| IBS file for GS832xxxxxA
| Package: standard 209pin BGA
| DQ driver is programmable
| VDD=3.3V, VDDQ can be either 2.5V or 3.3V
| Date:   23 August 2006
| Rev.:
[IBIS Ver]   3.2
[File name]   gs832xxxxxa.ibs
[File Rev]   1.0
[Date]   08/23/06
[Component]   GS832018T
[Manufacturer]   GSI Technology
[Package]
|  variable   typ   min   max
R_pkg   0.2   0.1   0.5
L_pkg   3nH   1nH   5nH
C_pkg   1.5pF   1pF   3pF
[Pin]   signal_name model_name  R_pin   L_pin   C_pin
 1   NC   NC
 2   NC   NC
 3   NC   NC
 4   VDDQ   POWER
 5   VSS   GND
 6   NC   NC
 7   NC   NC
 8   DQB1   Progbuf1
 9   DQB2   Progbuf1
 10   VSS   GND
 11   VDDQ   POWER
 12   DQB3   Progbuf1
 13   DQB4   Progbuf1
 14   FT#   INBUF
 15   VDD   POWER
 16   NC   NC
 17   VSS   GND
 18   DQB5   Progbuf1
 19   DQB6   Progbuf1
 20   VDDQ   POWER
 21   VSS   GND
 22   DQB7   Progbuf1
 23   DQB8   Progbuf1
 24   DQB9   Progbuf1
 25   NC   NC
 26   VSS   GND
 27   VDDQ   POWER
 28   NC   NC
 29   NC   NC
 30   NC   NC
 31   LBO#   INBUF
 32   A5   INBUF
 33   A4   INBUF
 34   A3   INBUF
 35   A2   INBUF
 36   A1   INBUF
 37   A0   INBUF
 38   NC   NC
 39   A19   INBUF
 40   VSS   GND
 41   VDD   POWER
 42   A18   INBUF
 43   A17   INBUF
 44   A10   INBUF
 45   A11   INBUF
 46   A12   INBUF
 47   A13   INBUF
 48   A14   INBUF
 49   A15   INBUF
 50   A16   INBUF
 51   NC   NC
 52   NC   NC
 53   NC   NC
 54   VDDQ   POWER
 55   VSS   GND
 56   NC   NC
 57   NC   NC
 58   DQA1   Progbuf1
 59   DQA2   Progbuf1
 60   VSS   GND
 61   VDDQ   POWER
 62   DQA3   Progbuf1
 63   DQA4   Progbuf1
 64   ZZ   INBUF
 65   VDD   POWER
 66   NC   NC
 67   VSS   GND
 68   DQA5   Progbuf1
 69   DQA6   Progbuf1
 70   VDDQ   POWER
 71   VSS   GND
 72   DQA7   Progbuf1
 73   DQA8   Progbuf1
 74   DQA9   Progbuf1
 75   NC   NC
 76   VSS   GND
 77   VDDQ   POWER
 78   NC   NC
 79   NC   NC
 80   A20   INBUF
 81   A9   INBUF
 82   A8   INBUF
 83   ADV#   INBUF
 84   ADSP#   INBUF
 85   ADSC#   INBUF
 86   G#   INBUF
 87   BW#   INBUF
 88   GW#   INBUF
 89   CK   INBUF
 90   VSS   GND
 91   VDD   POWER
 92   E3#   INBUF
 93   BA#   INBUF
 94   BB#   INBUF
 95   NC   NC
 96   NC   NC
 97   E2   INBUF
 98   E1#   INBUF
 99   A7   INBUF
 100   A6   INBUF
[Component]   GS832032T
[Manufacturer]   GSI Technology
[Package]
|  variable   typ   min   max
R_pkg   0.2   0.1   0.5
L_pkg   3nH   1nH   5nH
C_pkg   1.5pF   1pF   3pF
[Pin]   signal_name model_name  R_pin   L_pin   C_pin
 1   NC   NC
 2   DQC8   Progbuf1
 3   DQC7   Progbuf1
 4   VDDQ   POWER
 5   VSS   GND
 6   DQC6   Progbuf1
 7   DQC5   Progbuf1
 8   DQC4   Progbuf1
 9   DQC3   Progbuf1
 10   VSS   GND
 11   VDDQ   POWER
 12   DQC2   Progbuf1
 13   DQC1   Progbuf1
 14   FT#   INBUF
 15   VDD   POWER
 16   NC   NC
 17   VSS   GND
 18   DQD1   Progbuf1
 19   DQD2   Progbuf1
 20   VDDQ   POWER
 21   VSS   GND
 22   DQD3   Progbuf1
 23   DQD4   Progbuf1
 24   DQD5   Progbuf1
 25   DQD6   Progbuf1
 26   VSS   GND
 27   VDDQ   POWER
 28   DQD7   Progbuf1
 29   DQD8   Progbuf1
 30   NC   NC
 31   LBO#   INBUF
 32   A5   INBUF
 33   A4   INBUF
 34   A3   INBUF
 35   A2   INBUF
 36   A1   INBUF
 37   A0   INBUF
 38   NC   NC
 39   A19   INBUF
 40   VSS   GND
 41   VDD   POWER
 42   A18   INBUF
 43   A17   INBUF
 44   A10   INBUF
 45   A11   INBUF
 46   A12   INBUF
 47   A13   INBUF
 48   A14   INBUF
 49   A15   INBUF
 50   A16   INBUF
 51   NC   NC
 52   DQA8   Progbuf1
 53   DQA7   Progbuf1
 54   VDDQ   POWER
 55   VSS   GND
 56   DQA6   Progbuf1
 57   DQA5   Progbuf1
 58   DQA4   Progbuf1
 59   DQA3   Progbuf1
 60   VSS   GND
 61   VDDQ   POWER
 62   DQA2   Progbuf1
 63   DQA1   Progbuf1
 64   ZZ   INBUF
 65   VDD   POWER
 66   NC   NC
 67   VSS   GND
 68   DQB1   Progbuf1
 69   DQB2   Progbuf1
 70   VDDQ   POWER
 71   VSS   GND
 72   DQB3   Progbuf1
 73   DQB4   Progbuf1
 74   DQB5   Progbuf1
 75   DQB6   Progbuf1
 76   VSS   GND
 77   VDDQ   POWER
 78   DQB7   Progbuf1
 79   DQB8   Progbuf1
 80   NC   NC
 81   A9   INBUF
 82   A8   INBUF
 83   ADV#   INBUF
 84   ADSP#   INBUF
 85   ADSC#   INBUF
 86   G#   INBUF
 87   BW#   INBUF
 88   GW#   INBUF
 89   CK   INBUF
 90   VSS   GND
 91   VDD   POWER
 92   E3#   INBUF
 93   BA#   INBUF
 94   BB#   INBUF
 95   BC#   INBUF
 96   BD#   INBUF
 97   E2   INBUF
 98   E1#   INBUF
 99   A7   INBUF
 100   A6   INBUF
[Component]   GS832036T
[Manufacturer]   GSI Technology
[Package]
|  variable   typ   min   max
R_pkg   0.2   0.1   0.5
L_pkg   3nH   1nH   5nH
C_pkg   1.5pF   1pF   3pF
[Pin]   signal_name model_name  R_pin   L_pin   C_pin
 1   DQC9   Progbuf1
 2   DQC8   Progbuf1
 3   DQC7   Progbuf1
 4   VDDQ   POWER
 5   VSS   GND
 6   DQC6   Progbuf1
 7   DQC5   Progbuf1
 8   DQC4   Progbuf1
 9   DQC3   Progbuf1
 10   VSS   GND
 11   VDDQ   POWER
 12   DQC2   Progbuf1
 13   DQC1   Progbuf1
 14   FT#   INBUF
 15   VDD   POWER
 16   NC   NC
 17   VSS   GND
 18   DQD1   Progbuf1
 19   DQD2   Progbuf1
 20   VDDQ   POWER
 21   VSS   GND
 22   DQD3   Progbuf1
 23   DQD4   Progbuf1
 24   DQD5   Progbuf1
 25   DQD6   Progbuf1
 26   VSS   GND
 27   VDDQ   POWER
 28   DQD7   Progbuf1
 29   DQD8   Progbuf1
 30   DQD9   Progbuf1
 31   LBO#   INBUF
 32   A5   INBUF
 33   A4   INBUF
 34   A3   INBUF
 35   A2   INBUF
 36   A1   INBUF
 37   A0   INBUF
 38   NC   NC
 39   A19   INBUF
 40   VSS   GND
 41   VDD   POWER
 42   A18   INBUF
 43   A17   INBUF
 44   A10   INBUF
 45   A11   INBUF
 46   A12   INBUF
 47   A13   INBUF
 48   A14   INBUF
 49   A15   INBUF
 50   A16   INBUF
 51   DQA9   Progbuf1
 52   DQA8   Progbuf1
 53   DQA7   Progbuf1
 54   VDDQ   POWER
 55   VSS   GND
 56   DQA6   Progbuf1
 57   DQA5   Progbuf1
 58   DQA4   Progbuf1
 59   DQA3   Progbuf1
 60   VSS   GND
 61   VDDQ   POWER
 62   DQA2   Progbuf1
 63   DQA1   Progbuf1
 64   ZZ   INBUF
 65   VDD   POWER
 66   NC   NC
 67   VSS   GND
 68   DQB1   Progbuf1
 69   DQB2   Progbuf1
 70   VDDQ   POWER
 71   VSS   GND
 72   DQB3   Progbuf1
 73   DQB4   Progbuf1
 74   DQB5   Progbuf1
 75   DQB6   Progbuf1
 76   VSS   GND
 77   VDDQ   POWER
 78   DQB7   Progbuf1
 79   DQB8   Progbuf1
 80   DQB9   Progbuf1
 81   A9   INBUF
 82   A8   INBUF
 83   ADV#   INBUF
 84   ADSP#   INBUF
 85   ADSC#   INBUF
 86   G#   INBUF
 87   BW#   INBUF
 88   GW#   INBUF
 89   CK   INBUF
 90   VSS   GND
 91   VDD   POWER
 92   E3#   INBUF
 93   BA#   INBUF
 94   BB#   INBUF
 95   BC#   INBUF
 96   BD#   INBUF
 97   E2   INBUF
 98   E1#   INBUF
 99   A7   INBUF
 100   A6   INBUF
[Component]   GS8320e18T
[Manufacturer]   GSI Technology
[Package]
|  variable   typ   min   max
R_pkg   0.2   0.1   0.5
L_pkg   3nH   1nH   5nH
C_pkg   1.5pF   1pF   3pF
[Pin]   signal_name model_name  R_pin   L_pin   C_pin
 1   NC   NC
 2   NC   NC
 3   NC   NC
 4   VDDQ   POWER
 5   VSS   GND
 6   NC   NC
 7   NC   NC
 8   DQB1   Progbuf1
 9   DQB2   Progbuf1
 10   VSS   GND
 11   VDDQ   POWER
 12   DQB3   Progbuf1
 13   DQB4   Progbuf1
 14   FT#   INBUF
 15   VDD   POWER
 16   NC   NC
 17   VSS   GND
 18   DQB5   Progbuf1
 19   DQB6   Progbuf1
 20   VDDQ   POWER
 21   VSS   GND
 22   DQB7   Progbuf1
 23   DQB8   Progbuf1
 24   DQB9   Progbuf1
 25   NC   NC
 26   VSS   GND
 27   VDDQ   POWER
 28   NC   NC
 29   NC   NC
 30   NC   NC
 31   LBO#   INBUF
 32   A5   INBUF
 33   A4   INBUF
 34   A3   INBUF
 35   A2   INBUF
 36   A1   INBUF
 37   A0   INBUF
 38   NC   NC
 39   A19   INBUF
 40   VSS   GND
 41   VDD   POWER
 42   A18   INBUF
 43   A17   INBUF
 44   A10   INBUF
 45   A11   INBUF
 46   A12   INBUF
 47   A13   INBUF
 48   A14   INBUF
 49   A15   INBUF
 50   A16   INBUF
 51   NC   NC
 52   NC   NC
 53   NC   NC
 54   VDDQ   POWER
 55   VSS   GND
 56   NC   NC
 57   NC   NC
 58   DQA1   Progbuf1
 59   DQA2   Progbuf1
 60   VSS   GND
 61   VDDQ   POWER
 62   DQA3   Progbuf1
 63   DQA4   Progbuf1
 64   ZZ   INBUF
 65   VDD   POWER
 66   NC   NC
 67   VSS   GND
 68   DQA5   Progbuf1
 69   DQA6   Progbuf1
 70   VDDQ   POWER
 71   VSS   GND
 72   DQA7   Progbuf1
 73   DQA8   Progbuf1
 74   DQA9   Progbuf1
 75   NC   NC
 76   VSS   GND
 77   VDDQ   POWER
 78   NC   NC
 79   NC   NC
 80   A20   INBUF
 81   A9   INBUF
 82   A8   INBUF
 83   ADV#   INBUF
 84   ADSP#   INBUF
 85   ADSC#   INBUF
 86   G#   INBUF
 87   BW#   INBUF
 88   GW#   INBUF
 89   CK   INBUF
 90   VSS   GND
 91   VDD   POWER
 92   E3#   INBUF
 93   BA#   INBUF
 94   BB#   INBUF
 95   NC   NC
 96   NC   NC
 97   E2   INBUF
 98   E1#   INBUF
 99   A7   INBUF
 100   A6   INBUF
[Component]   GS8320e32T
[Manufacturer]   GSI Technology
[Package]
|  variable   typ   min   max
R_pkg   0.2   0.1   0.5
L_pkg   3nH   1nH   5nH
C_pkg   1.5pF   1pF   3pF
[Pin]   signal_name model_name  R_pin   L_pin   C_pin
 1   NC   NC
 2   DQC8   Progbuf1
 3   DQC7   Progbuf1
 4   VDDQ   POWER
 5   VSS   GND
 6   DQC6   Progbuf1
 7   DQC5   Progbuf1
 8   DQC4   Progbuf1
 9   DQC3   Progbuf1
 10   VSS   GND
 11   VDDQ   POWER
 12   DQC2   Progbuf1
 13   DQC1   Progbuf1
 14   FT#   INBUF
 15   VDD   POWER
 16   NC   NC
 17   VSS   GND
 18   DQD1   Progbuf1
 19   DQD2   Progbuf1
 20   VDDQ   POWER
 21   VSS   GND
 22   DQD3   Progbuf1
 23   DQD4   Progbuf1
 24   DQD5   Progbuf1
 25   DQD6   Progbuf1
 26   VSS   GND
 27   VDDQ   POWER
 28   DQD7   Progbuf1
 29   DQD8   Progbuf1
 30   NC   NC
 31   LBO#   INBUF
 32   A5   INBUF
 33   A4   INBUF
 34   A3   INBUF
 35   A2   INBUF
 36   A1   INBUF
 37   A0   INBUF
 38   NC   NC
 39   A19   INBUF
 40   VSS   GND
 41   VDD   POWER
 42   A18   INBUF
 43   A17   INBUF
 44   A10   INBUF
 45   A11   INBUF
 46   A12   INBUF
 47   A13   INBUF
 48   A14   INBUF
 49   A15   INBUF
 50   A16   INBUF
 51   NC   NC
 52   DQA8   Progbuf1
 53   DQA7   Progbuf1
 54   VDDQ   POWER
 55   VSS   GND
 56   DQA6   Progbuf1
 57   DQA5   Progbuf1
 58   DQA4   Progbuf1
 59   DQA3   Progbuf1
 60   VSS   GND
 61   VDDQ   POWER
 62   DQA2   Progbuf1
 63   DQA1   Progbuf1
 64   ZZ   INBUF
 65   VDD   POWER
 66   NC   NC
 67   VSS   GND
 68   DQB1   Progbuf1
 69   DQB2   Progbuf1
 70   VDDQ   POWER
 71   VSS   GND
 72   DQB3   Progbuf1
 73   DQB4   Progbuf1
 74   DQB5   Progbuf1
 75   DQB6   Progbuf1
 76   VSS   GND
 77   VDDQ   POWER
 78   DQB7   Progbuf1
 79   DQB8   Progbuf1
 80   NC   NC
 81   A9   INBUF
 82   A8   INBUF
 83   ADV#   INBUF
 84   ADSP#   INBUF
 85   ADSC#   INBUF
 86   G#   INBUF
 87   BW#   INBUF
 88   GW#   INBUF
 89   CK   INBUF
 90   VSS   GND
 91   VDD   POWER
 92   E3#   INBUF
 93   BA#   INBUF
 94   BB#   INBUF
 95   BC#   INBUF
 96   BD#   INBUF
 97   E2   INBUF
 98   E1#   INBUF
 99   A7   INBUF
 100   A6   INBUF
[Component]   GS8320e36T
[Manufacturer]   GSI Technology
[Package]
|  variable   typ   min   max
R_pkg   0.2   0.1   0.5
L_pkg   3nH   1nH   5nH
C_pkg   1.5pF   1pF   3pF
[Pin]   signal_name model_name  R_pin   L_pin   C_pin
 1   DQC9   Progbuf1
 2   DQC8   Progbuf1
 3   DQC7   Progbuf1
 4   VDDQ   POWER
 5   VSS   GND
 6   DQC6   Progbuf1
 7   DQC5   Progbuf1
 8   DQC4   Progbuf1
 9   DQC3   Progbuf1
 10   VSS   GND
 11   VDDQ   POWER
 12   DQC2   Progbuf1
 13   DQC1   Progbuf1
 14   FT#   INBUF
 15   VDD   POWER
 16   NC   NC
 17   VSS   GND
 18   DQD1   Progbuf1
 19   DQD2   Progbuf1
 20   VDDQ   POWER
 21   VSS   GND
 22   DQD3   Progbuf1
 23   DQD4   Progbuf1
 24   DQD5   Progbuf1
 25   DQD6   Progbuf1
 26   VSS   GND
 27   VDDQ   POWER
 28   DQD7   Progbuf1
 29   DQD8   Progbuf1
 30   DQD9   Progbuf1
 31   LBO#   INBUF
 32   A5   INBUF
 33   A4   INBUF
 34   A3   INBUF
 35   A2   INBUF
 36   A1   INBUF
 37   A0   INBUF
 38   NC   NC
 39   A19   INBUF
 40   VSS   GND
 41   VDD   POWER
 42   A18   INBUF
 43   A17   INBUF
 44   A10   INBUF
 45   A11   INBUF
 46   A12   INBUF
 47   A13   INBUF
 48   A14   INBUF
 49   A15   INBUF
 50   A16   INBUF
 51   DQA9   Progbuf1
 52   DQA8   Progbuf1
 53   DQA7   Progbuf1
 54   VDDQ   POWER
 55   VSS   GND
 56   DQA6   Progbuf1
 57   DQA5   Progbuf1
 58   DQA4   Progbuf1
 59   DQA3   Progbuf1
 60   VSS   GND
 61   VDDQ   POWER
 62   DQA2   Progbuf1
 63   DQA1   Progbuf1
 64   ZZ   INBUF
 65   VDD   POWER
 66   NC   NC
 67   VSS   GND
 68   DQB1   Progbuf1
 69   DQB2   Progbuf1
 70   VDDQ   POWER
 71   VSS   GND
 72   DQB3   Progbuf1
 73   DQB4   Progbuf1
 74   DQB5   Progbuf1
 75   DQB6   Progbuf1
 76   VSS   GND
 77   VDDQ   POWER
 78   DQB7   Progbuf1
 79   DQB8   Progbuf1
 80   DQB9   Progbuf1
 81   A9   INBUF
 82   A8   INBUF
 83   ADV#   INBUF
 84   ADSP#   INBUF
 85   ADSC#   INBUF
 86   G#   INBUF
 87   BW#   INBUF
 88   GW#   INBUF
 89   CK   INBUF
 90   VSS   GND
 91   VDD   POWER
 92   E3#   INBUF
 93   BA#   INBUF
 94   BB#   INBUF
 95   BC#   INBUF
 96   BD#   INBUF
 97   E2   INBUF
 98   E1#   INBUF
 99   A7   INBUF
 100   A6   INBUF
[Component]   GS8320f18T
[Manufacturer]   GSI Technology
[Package]
|  variable   typ   min   max
R_pkg   0.2   0.1   0.5
L_pkg   3nH   1nH   5nH
C_pkg   1.5pF   1pF   3pF
[Pin]   signal_name model_name  R_pin   L_pin   C_pin
 1   NC   NC
 2   NC   NC
 3   NC   NC
 4   VDDQ   POWER
 5   VSS   GND
 6   NC   NC
 7   NC   NC
 8   DQB1   Progbuf1
 9   DQB2   Progbuf1
 10   VSS   GND
 11   VDDQ   POWER
 12   DQB3   Progbuf1
 13   DQB4   Progbuf1
 14   NC   NC
 15   VDD   POWER
 16   NC   NC
 17   VSS   GND
 18   DQB5   Progbuf1
 19   DQB6   Progbuf1
 20   VDDQ   POWER
 21   VSS   GND
 22   DQB7   Progbuf1
 23   DQB8   Progbuf1
 24   DQB9   Progbuf1
 25   NC   NC
 26   VSS   GND
 27   VDDQ   POWER
 28   NC   NC
 29   NC   NC
 30   NC   NC
 31   LBO#   INBUF
 32   A5   INBUF
 33   A4   INBUF
 34   A3   INBUF
 35   A2   INBUF
 36   A1   INBUF
 37   A0   INBUF
 38   NC   NC
 39   A19   INBUF
 40   VSS   GND
 41   VDD   POWER
 42   A18   INBUF
 43   A17   INBUF
 44   A10   INBUF
 45   A11   INBUF
 46   A12   INBUF
 47   A13   INBUF
 48   A14   INBUF
 49   A15   INBUF
 50   A16   INBUF
 51   NC   NC
 52   NC   NC
 53   NC   NC
 54   VDDQ   POWER
 55   VSS   GND
 56   NC   NC
 57   NC   NC
 58   DQA1   Progbuf1
 59   DQA2   Progbuf1
 60   VSS   GND
 61   VDDQ   POWER
 62   DQA3   Progbuf1
 63   DQA4   Progbuf1
 64   ZZ   INBUF
 65   VDD   POWER
 66   NC   NC
 67   VSS   GND
 68   DQA5   Progbuf1
 69   DQA6   Progbuf1
 70   VDDQ   POWER
 71   VSS   GND
 72   DQA7   Progbuf1
 73   DQA8   Progbuf1
 74   DQA9   Progbuf1
 75   NC   NC
 76   VSS   GND
 77   VDDQ   POWER
 78   NC   NC
 79   NC   NC
 80   A20   INBUF
 81   A9   INBUF
 82   A8   INBUF
 83   ADV#   INBUF
 84   ADSP#   INBUF
 85   ADSC#   INBUF
 86   G#   INBUF
 87   BW#   INBUF
 88   GW#   INBUF
 89   CK   INBUF
 90   VSS   GND
 91   VDD   POWER
 92   E3#   INBUF
 93   BA#   INBUF
 94   BB#   INBUF
 95   NC   NC
 96   NC   NC
 97   E2   INBUF
 98   E1#   INBUF
 99   A7   INBUF
 100   A6   INBUF
[Component]   GS8320f32T
[Manufacturer]   GSI Technology
[Package]
|  variable   typ   min   max
R_pkg   0.2   0.1   0.5
L_pkg   3nH   1nH   5nH
C_pkg   1.5pF   1pF   3pF
[Pin]   signal_name model_name  R_pin   L_pin   C_pin
 1   NC   NC
 2   DQC8   Progbuf1
 3   DQC7   Progbuf1
 4   VDDQ   POWER
 5   VSS   GND
 6   DQC6   Progbuf1
 7   DQC5   Progbuf1
 8   DQC4   Progbuf1
 9   DQC3   Progbuf1
 10   VSS   GND
 11   VDDQ   POWER
 12   DQC2   Progbuf1
 13   DQC1   Progbuf1
 14   NC   NC
 15   VDD   POWER
 16   NC   NC
 17   VSS   GND
 18   DQD1   Progbuf1
 19   DQD2   Progbuf1
 20   VDDQ   POWER
 21   VSS   GND
 22   DQD3   Progbuf1
 23   DQD4   Progbuf1
 24   DQD5   Progbuf1
 25   DQD6   Progbuf1
 26   VSS   GND
 27   VDDQ   POWER
 28   DQD7   Progbuf1
 29   DQD8   Progbuf1
 30   NC   NC
 31   LBO#   INBUF
 32   A5   INBUF
 33   A4   INBUF
 34   A3   INBUF
 35   A2   INBUF
 36   A1   INBUF
 37   A0   INBUF
 38   NC   NC
 39   A19   INBUF
 40   VSS   GND
 41   VDD   POWER
 42   A18   INBUF
 43   A17   INBUF
 44   A10   INBUF
 45   A11   INBUF
 46   A12   INBUF
 47   A13   INBUF
 48   A14   INBUF
 49   A15   INBUF
 50   A16   INBUF
 51   NC   NC
 52   DQA8   Progbuf1
 53   DQA7   Progbuf1
 54   VDDQ   POWER
 55   VSS   GND
 56   DQA6   Progbuf1
 57   DQA5   Progbuf1
 58   DQA4   Progbuf1
 59   DQA3   Progbuf1
 60   VSS   GND
 61   VDDQ   POWER
 62   DQA2   Progbuf1
 63   DQA1   Progbuf1
 64   ZZ   INBUF
 65   VDD   POWER
 66   NC   NC
 67   VSS   GND
 68   DQB1   Progbuf1
 69   DQB2   Progbuf1
 70   VDDQ   POWER
 71   VSS   GND
 72   DQB3   Progbuf1
 73   DQB4   Progbuf1
 74   DQB5   Progbuf1
 75   DQB6   Progbuf1
 76   VSS   GND
 77   VDDQ   POWER
 78   DQB7   Progbuf1
 79   DQB8   Progbuf1
 80   NC   NC
 81   A9   INBUF
 82   A8   INBUF
 83   ADV#   INBUF
 84   ADSP#   INBUF
 85   ADSC#   INBUF
 86   G#   INBUF
 87   BW#   INBUF
 88   GW#   INBUF
 89   CK   INBUF
 90   VSS   GND
 91   VDD   POWER
 92   E3#   INBUF
 93   BA#   INBUF
 94   BB#   INBUF
 95   BC#   INBUF
 96   BD#   INBUF
 97   E2   INBUF
 98   E1#   INBUF
 99   A7   INBUF
 100   A6   INBUF
[Component]   GS8320f36T
[Manufacturer]   GSI Technology
[Package]
|  variable   typ   min   max
R_pkg   0.2   0.1   0.5
L_pkg   3nH   1nH   5nH
C_pkg   1.5pF   1pF   3pF
[Pin]   signal_name model_name  R_pin   L_pin   C_pin
 1   DQC9   Progbuf1
 2   DQC8   Progbuf1
 3   DQC7   Progbuf1
 4   VDDQ   POWER
 5   VSS   GND
 6   DQC6   Progbuf1
 7   DQC5   Progbuf1
 8   DQC4   Progbuf1
 9   DQC3   Progbuf1
 10   VSS   GND
 11   VDDQ   POWER
 12   DQC2   Progbuf1
 13   DQC1   Progbuf1
 14   NC   NC
 15   VDD   POWER
 16   NC   NC
 17   VSS   GND
 18   DQD1   Progbuf1
 19   DQD2   Progbuf1
 20   VDDQ   POWER
 21   VSS   GND
 22   DQD3   Progbuf1
 23   DQD4   Progbuf1
 24   DQD5   Progbuf1
 25   DQD6   Progbuf1
 26   VSS   GND
 27   VDDQ   POWER
 28   DQD7   Progbuf1
 29   DQD8   Progbuf1
 30   DQD9   Progbuf1
 31   LBO#   INBUF
 32   A5   INBUF
 33   A4   INBUF
 34   A3   INBUF
 35   A2   INBUF
 36   A1   INBUF
 37   A0   INBUF
 38   NC   NC
 39   A19   INBUF
 40   VSS   GND
 41   VDD   POWER
 42   A18   INBUF
 43   A17   INBUF
 44   A10   INBUF
 45   A11   INBUF
 46   A12   INBUF
 47   A13   INBUF
 48   A14   INBUF
 49   A15   INBUF
 50   A16   INBUF
 51   DQA9   Progbuf1
 52   DQA8   Progbuf1
 53   DQA7   Progbuf1
 54   VDDQ   POWER
 55   VSS   GND
 56   DQA6   Progbuf1
 57   DQA5   Progbuf1
 58   DQA4   Progbuf1
 59   DQA3   Progbuf1
 60   VSS   GND
 61   VDDQ   POWER
 62   DQA2   Progbuf1
 63   DQA1   Progbuf1
 64   ZZ   INBUF
 65   VDD   POWER
 66   NC   NC
 67   VSS   GND
 68   DQB1   Progbuf1
 69   DQB2   Progbuf1
 70   VDDQ   POWER
 71   VSS   GND
 72   DQB3   Progbuf1
 73   DQB4   Progbuf1
 74   DQB5   Progbuf1
 75   DQB6   Progbuf1
 76   VSS   GND
 77   VDDQ   POWER
 78   DQB7   Progbuf1
 79   DQB8   Progbuf1
 80   DQB9   Progbuf1
 81   A9   INBUF
 82   A8   INBUF
 83   ADV#   INBUF
 84   ADSP#   INBUF
 85   ADSC#   INBUF
 86   G#   INBUF
 87   BW#   INBUF
 88   GW#   INBUF
 89   CK   INBUF
 90   VSS   GND
 91   VDD   POWER
 92   E3#   INBUF
 93   BA#   INBUF
 94   BB#   INBUF
 95   BC#   INBUF
 96   BD#   INBUF
 97   E2   INBUF
 98   E1#   INBUF
 99   A7   INBUF
 100   A6   INBUF
[Component]   GS832118E
[Manufacturer]   GSI Technology
[Package]
|  variable   typ   min   max
R_pkg   0.2   0.1   0.5
L_pkg   3nH   1nH   5nH
C_pkg   1.5pF   1pF   3pF
[Pin]   signal_name model_name  R_pin   L_pin   C_pin
 A1   NC   NC
 A2   A14   INBUF
 A3   E1#   INBUF
 A4   BB#   INBUF
 A5   NC   NC
 A6   E3#   INBUF
 A7   BW#   INBUF
 A8   ADSC#   INBUF
 A9   ADV#   INBUF
 A10   A13   INBUF
 A11   A20   INBUF
 B1   NC   NC
 B2   A16   INBUF
 B3   E2   INBUF
 B4   NC   NC
 B5   BA#   INBUF
 B6   CK   INBUF
 B7   GW#   INBUF
 B8   G#   INBUF
 B9   ADSP   INBUF
 B10   A15   INBUF
 B11   NC   NC
 C1   NC   NC
 C2   NC   NC
 C3   VDDQ   POWER
 C4   VSS   GND
 C5   VSS   GND
 C6   VSS   GND
 C7   VSS   GND
 C8   VSS   GND
 C9   VDDQ   POWER
 C10   NC   NC
 C11   DQPA   Progbuf1
 D1   NC   NC
 D2   DQB1   Progbuf1
 D3   VDDQ   POWER
 D4   VDD   POWER
 D5   VSS   GND
 D6   VSS   GND
 D7   VSS   GND
 D8   VDD   POWER
 D9   VDDQ   POWER
 D10   NC   NC
 D11   DQA8   Progbuf1
 E1   NC   NC
 E2   DQB2   Progbuf1
 E3   VDDQ   POWER
 E4   VDD   POWER
 E5   VSS   GND
 E6   VSS   GND
 E7   VSS   GND
 E8   VDD   POWER
 E9   VDDQ   POWER
 E10   NC   NC
 E11   DQA7   Progbuf1
 F1   NC   NC
 F2   DQB3   Progbuf1
 F3   VDDQ   POWER
 F4   VDD   POWER
 F5   VSS   GND
 F6   VSS   GND
 F7   VSS   GND
 F8   VDD   POWER
 F9   VDDQ   POWER
 F10   NC   NC
 F11   DQA6   Progbuf1
 G1   NC   NC
 G2   DQB4   Progbuf1
 G3   VDDQ   POWER
 G4   VDD   POWER
 G5   VSS   GND
 G6   VSS   GND
 G7   VSS   GND
 G8   VDD   POWER
 G9   VDDQ   POWER
 G10   NC   NC
 G11   DQA5   Progbuf1
 H1   FT#   INBUF
 H2   MCL   INBUF
 H3   NC   NC
 H4   VDD   POWER
 H5   VSS   GND
 H6   VSS   GND
 H7   VSS   GND
 H8   VDD   POWER
 H9   NC   NC
 H10   NC   NC
 H11   ZZ   INBUF
 J1   DQB5   Progbuf1
 J2   NC   NC
 J3   VDDQ   POWER
 J4   VDD   POWER
 J5   VSS   GND
 J6   VSS   GND
 J7   VSS   GND
 J8   VDD   POWER
 J9   VDDQ   POWER
 J10   DQA4   Progbuf1
 J11   NC   NC
 K1   DQB6   Progbuf1
 K2   NC   NC
 K3   VDDQ   POWER
 K4   VDD   POWER
 K5   VSS   GND
 K6   VSS   GND
 K7   VSS   GND
 K8   VDD   POWER
 K9   VDDQ   POWER
 K10   DQA3   Progbuf1
 K11   NC   NC
 L1   DQB7   Progbuf1
 L2   NC   NC
 L3   VDDQ   POWER
 L4   VDD   POWER
 L5   VSS   GND
 L6   VSS   GND
 L7   VSS   GND
 L8   VDD   POWER
 L9   VDDQ   POWER
 L10   DQA2   Progbuf1
 L11   NC   NC
 M1   DQB8   Progbuf1
 M2   NC   NC
 M3   VDDQ   POWER
 M4   VDD   POWER
 M5   VSS   GND
 M6   VSS   GND
 M7   VSS   GND
 M8   VDD   POWER
 M9   VDDQ   POWER
 M10   DQA1   Progbuf1
 M11   NC   NC
 N1   DQPB   Progbuf1
 N2   SCD   INBUF
 N3   VDDQ   POWER
 N4   VSS   GND
 N5   NC   NC
 N6   A18   INBUF
 N7   NC   NC
 N8   VSS   GND
 N9   VDDQ   POWER
 N10   NC   NC
 N11   NC   NC
 P1   NC   NC
 P2   NC   NC
 P3   A6   INBUF
 P4   A5   INBUF
 P5   TDI   INBUF
 P6   A1   INBUF
 P7   TDO   Progbuf2
 P8   A4   INBUF
 P9   A3   INBUF
 P10   A2   INBUF
 P11   A17   INBUF
 R1   LBO#   INBUF
 R2   A19   INBUF
 R3   A12   INBUF
 R4   A11   INBUF
 R5   TMS   INBUF
 R6   A0   INBUF
 R7   TCK   INBUF
 R8   A10   INBUF
 R9   A9   INBUF
 R10   A8   INBUF
 R11   A7   INBUF
[Component]   GS832132E
[Manufacturer]   GSI Technology
[Package]
|  variable   typ   min   max
R_pkg   0.2   0.1   0.5
L_pkg   3nH   1nH   5nH
C_pkg   1.5pF   1pF   3pF
[Pin]   signal_name model_name  R_pin   L_pin   C_pin
 A1   NC   NC
 A2   A14   INBUF
 A3   E1#   INBUF
 A4   BC#   INBUF
 A5   BB#   INBUF
 A6   E3#   INBUF
 A7   BW#   INBUF
 A8   ADSC#   INBUF
 A9   ADV#   INBUF
 A10   A13   INBUF
 A11   NC   NC
 B1   NC   NC
 B2   A16   INBUF
 B3   E2   INBUF
 B4   BD#   INBUF
 B5   BA#   INBUF
 B6   CK   INBUF
 B7   GW#   INBUF
 B8   G#   INBUF
 B9   ADSP   INBUF
 B10   A15   INBUF
 B11   NC   NC
 C1   NC   NC
 C2   NC   NC
 C3   VDDQ   POWER
 C4   VSS   GND
 C5   VSS   GND
 C6   VSS   GND
 C7   VSS   GND
 C8   VSS   GND
 C9   VDDQ   POWER
 C10   NC   NC
 C11   NC   NC
 D1   DQC8   Progbuf1
 D2   DQC4   Progbuf1
 D3   VDDQ   POWER
 D4   VDD   POWER
 D5   VSS   GND
 D6   VSS   GND
 D7   VSS   GND
 D8   VDD   POWER
 D9   VDDQ   POWER
 D10   DQB4   Progbuf1
 D11   DQB8   Progbuf1
 E1   DQC7   Progbuf1
 E2   DQC3   Progbuf1
 E3   VDDQ   POWER
 E4   VDD   POWER
 E5   VSS   GND
 E6   VSS   GND
 E7   VSS   GND
 E8   VDD   POWER
 E9   VDDQ   POWER
 E10   DQB3   Progbuf1
 E11   DQB7   Progbuf1
 F1   DQC6   Progbuf1
 F2   DQC2   Progbuf1
 F3   VDDQ   POWER
 F4   VDD   POWER
 F5   VSS   GND
 F6   VSS   GND
 F7   VSS   GND
 F8   VDD   POWER
 F9   VDDQ   POWER
 F10   DQB2   Progbuf1
 F11   DQB6   Progbuf1
 G1   DQC5   Progbuf1
 G2   DQC1   Progbuf1
 G3   VDDQ   POWER
 G4   VDD   POWER
 G5   VSS   GND
 G6   VSS   GND
 G7   VSS   GND
 G8   VDD   POWER
 G9   VDDQ   POWER
 G10   DQB1   Progbuf1
 G11   DQB5   Progbuf1
 H1   FT#   INBUF
 H2   MCL   INBUF
 H3   NC   NC
 H4   VDD   POWER
 H5   VSS   GND
 H6   VSS   GND
 H7   VSS   GND
 H8   VDD   POWER
 H9   NC   NC
 H10   NC   NC
 H11   ZZ   INBUF
 J1   DQD5   Progbuf1
 J2   DQD1   Progbuf1
 J3   VDDQ   POWER
 J4   VDD   POWER
 J5   VSS   GND
 J6   VSS   GND
 J7   VSS   GND
 J8   VDD   POWER
 J9   VDDQ   POWER
 J10   DQA1   Progbuf1
 J11   DQA5   Progbuf1
 K1   DQD6   Progbuf1
 K2   DQD2   Progbuf1
 K3   VDDQ   POWER
 K4   VDD   POWER
 K5   VSS   GND
 K6   VSS   GND
 K7   VSS   GND
 K8   VDD   POWER
 K9   VDDQ   POWER
 K10   DQA2   Progbuf1
 K11   DQA6   Progbuf1
 L1   DQD7   Progbuf1
 L2   DQD3   Progbuf1
 L3   VDDQ   POWER
 L4   VDD   POWER
 L5   VSS   GND
 L6   VSS   GND
 L7   VSS   GND
 L8   VDD   POWER
 L9   VDDQ   POWER
 L10   DQA3   Progbuf1
 L11   DQA7   Progbuf1
 M1   DQD8   Progbuf1
 M2   DQD4   Progbuf1
 M3   VDDQ   POWER
 M4   VDD   POWER
 M5   VSS   GND
 M6   VSS   GND
 M7   VSS   GND
 M8   VDD   POWER
 M9   VDDQ   POWER
 M10   DQA4   Progbuf1
 M11   DQA8   Progbuf1
 N1   NC   NC
 N2   NC   NC
 N3   VDDQ   POWER
 N4   VSS   GND
 N5   NC   NC
 N6   A18   INBUF
 N7   NC   NC
 N8   VSS   GND
 N9   VDDQ   POWER
 N10   NC   NC
 N11   NC   NC
 P1   NC   NC
 P2   NC   NC
 P3   A6   INBUF
 P4   A5   INBUF
 P5   TDI   INBUF
 P6   A1   INBUF
 P7   TDO   Progbuf2
 P8   A4   INBUF
 P9   A3   INBUF
 P10   A2   INBUF
 P11   A17   INBUF
 R1   LBO#   INBUF
 R2   A19   INBUF
 R3   A12   INBUF
 R4   A11   INBUF
 R5   TMS   INBUF
 R6   A0   INBUF
 R7   TCK   INBUF
 R8   A10   INBUF
 R9   A9   INBUF
 R10   A8   INBUF
 R11   A7   INBUF
[Component]   GS832136E
[Manufacturer]   GSI Technology
[Package]
|  variable   typ   min   max
R_pkg   0.2   0.1   0.5
L_pkg   3nH   1nH   5nH
C_pkg   1.5pF   1pF   3pF
[Pin]   signal_name model_name  R_pin   L_pin   C_pin
 A1   NC   NC
 A2   A14   INBUF
 A3   E1#   INBUF
 A4   BC#   INBUF
 A5   BB#   INBUF
 A6   E3#   INBUF
 A7   BW#   INBUF
 A8   ADSC#   INBUF
 A9   ADV#   INBUF
 A10   A13   INBUF
 A11   NC   NC
 B1   NC   NC
 B2   A16   INBUF
 B3   E2   INBUF
 B4   BD#   INBUF
 B5   BA#   INBUF
 B6   CK   INBUF
 B7   GW#   INBUF
 B8   G#   INBUF
 B9   ADSP   INBUF
 B10   A15   INBUF
 B11   NC   NC
 C1   DQPC   Progbuf1
 C2   NC   NC
 C3   VDDQ   POWER
 C4   VSS   GND
 C5   VSS   GND
 C6   VSS   GND
 C7   VSS   GND
 C8   VSS   GND
 C9   VDDQ   POWER
 C10   NC   NC
 C11   DQPB   Progbuf1
 D1   DQC8   Progbuf1
 D2   DQC4   Progbuf1
 D3   VDDQ   POWER
 D4   VDD   POWER
 D5   VSS   GND
 D6   VSS   GND
 D7   VSS   GND
 D8   VDD   POWER
 D9   VDDQ   POWER
 D10   DQB4   Progbuf1
 D11   DQB8   Progbuf1
 E1   DQC7   Progbuf1
 E2   DQC3   Progbuf1
 E3   VDDQ   POWER
 E4   VDD   POWER
 E5   VSS   GND
 E6   VSS   GND
 E7   VSS   GND
 E8   VDD   POWER
 E9   VDDQ   POWER
 E10   DQB3   Progbuf1
 E11   DQB7   Progbuf1
 F1   DQC6   Progbuf1
 F2   DQC2   Progbuf1
 F3   VDDQ   POWER
 F4   VDD   POWER
 F5   VSS   GND
 F6   VSS   GND
 F7   VSS   GND
 F8   VDD   POWER
 F9   VDDQ   POWER
 F10   DQB2   Progbuf1
 F11   DQB6   Progbuf1
 G1   DQC5   Progbuf1
 G2   DQC1   Progbuf1
 G3   VDDQ   POWER
 G4   VDD   POWER
 G5   VSS   GND
 G6   VSS   GND
 G7   VSS   GND
 G8   VDD   POWER
 G9   VDDQ   POWER
 G10   DQB1   Progbuf1
 G11   DQB5   Progbuf1
 H1   FT#   INBUF
 H2   MCL   INBUF
 H3   NC   NC
 H4   VDD   POWER
 H5   VSS   GND
 H6   VSS   GND
 H7   VSS   GND
 H8   VDD   POWER
 H9   NC   NC
 H10   NC   NC
 H11   ZZ   INBUF
 J1   DQD5   Progbuf1
 J2   DQD1   Progbuf1
 J3   VDDQ   POWER
 J4   VDD   POWER
 J5   VSS   GND
 J6   VSS   GND
 J7   VSS   GND
 J8   VDD   POWER
 J9   VDDQ   POWER
 J10   DQA1   Progbuf1
 J11   DQA5   Progbuf1
 K1   DQD6   Progbuf1
 K2   DQD2   Progbuf1
 K3   VDDQ   POWER
 K4   VDD   POWER
 K5   VSS   GND
 K6   VSS   GND
 K7   VSS   GND
 K8   VDD   POWER
 K9   VDDQ   POWER
 K10   DQA2   Progbuf1
 K11   DQA6   Progbuf1
 L1   DQD7   Progbuf1
 L2   DQD3   Progbuf1
 L3   VDDQ   POWER
 L4   VDD   POWER
 L5   VSS   GND
 L6   VSS   GND
 L7   VSS   GND
 L8   VDD   POWER
 L9   VDDQ   POWER
 L10   DQA3   Progbuf1
 L11   DQA7   Progbuf1
 M1   DQD8   Progbuf1
 M2   DQD4   Progbuf1
 M3   VDDQ   POWER
 M4   VDD   POWER
 M5   VSS   GND
 M6   VSS   GND
 M7   VSS   GND
 M8   VDD   POWER
 M9   VDDQ   POWER
 M10   DQA4   Progbuf1
 M11   DQA8   Progbuf1
 N1   DQPD   Progbuf1
 N2   SCD   INBUF
 N3   VDDQ   POWER
 N4   VSS   GND
 N5   NC   NC
 N6   A18   INBUF
 N7   NC   NC
 N8   VSS   GND
 N9   VDDQ   POWER
 N10   NC   NC
 N11   DQPA   Progbuf1
 P1   NC   NC
 P2   NC   NC
 P3   A6   INBUF
 P4   A5   INBUF
 P5   TDI   INBUF
 P6   A1   INBUF
 P7   TDO   Progbuf2
 P8   A4   INBUF
 P9   A3   INBUF
 P10   A2   INBUF
 P11   A17   INBUF
 R1   LBO#   INBUF
 R2   A19   INBUF
 R3   A12   INBUF
 R4   A11   INBUF
 R5   TMS   INBUF
 R6   A0   INBUF
 R7   TCK   INBUF
 R8   A10   INBUF
 R9   A9   INBUF
 R10   A8   INBUF
 R11   A7   INBUF
[Component]   GS8321E18E
[Manufacturer]   GSI Technology
[Package]
|  variable   typ   min   max
R_pkg   0.2   0.1   0.5
L_pkg   3nH   1nH   5nH
C_pkg   1.5pF   1pF   3pF
[Pin]   signal_name model_name  R_pin   L_pin   C_pin
 A1   NC   NC
 A2   A14   INBUF
 A3   E1#   INBUF
 A4   BB#   INBUF
 A5   NC   NC
 A6   E3#   INBUF
 A7   BW#   INBUF
 A8   ADSC#   INBUF
 A9   ADV#   INBUF
 A10   A13   INBUF
 A11   A20   INBUF
 B1   NC   NC
 B2   A16   INBUF
 B3   E2   INBUF
 B4   NC   NC
 B5   BA#   INBUF
 B6   CK   INBUF
 B7   GW#   INBUF
 B8   G#   INBUF
 B9   ADSP   INBUF
 B10   A15   INBUF
 B11   NC   NC
 C1   NC   NC
 C2   NC   NC
 C3   VDDQ   POWER
 C4   VSS   GND
 C5   VSS   GND
 C6   VSS   GND
 C7   VSS   GND
 C8   VSS   GND
 C9   VDDQ   POWER
 C10   NC   NC
 C11   DQPA   Progbuf1
 D1   NC   NC
 D2   DQB1   Progbuf1
 D3   VDDQ   POWER
 D4   VDD   POWER
 D5   VSS   GND
 D6   VSS   GND
 D7   VSS   GND
 D8   VDD   POWER
 D9   VDDQ   POWER
 D10   NC   NC
 D11   DQA8   Progbuf1
 E1   NC   NC
 E2   DQB2   Progbuf1
 E3   VDDQ   POWER
 E4   VDD   POWER
 E5   VSS   GND
 E6   VSS   GND
 E7   VSS   GND
 E8   VDD   POWER
 E9   VDDQ   POWER
 E10   NC   NC
 E11   DQA7   Progbuf1
 F1   NC   NC
 F2   DQB3   Progbuf1
 F3   VDDQ   POWER
 F4   VDD   POWER
 F5   VSS   GND
 F6   VSS   GND
 F7   VSS   GND
 F8   VDD   POWER
 F9   VDDQ   POWER
 F10   NC   NC
 F11   DQA6   Progbuf1
 G1   NC   NC
 G2   DQB4   Progbuf1
 G3   VDDQ   POWER
 G4   VDD   POWER
 G5   VSS   GND
 G6   VSS   GND
 G7   VSS   GND
 G8   VDD   POWER
 G9   VDDQ   POWER
 G10   NC   NC
 G11   DQA5   Progbuf1
 H1   FT#   INBUF
 H2   MCL   INBUF
 H3   NC   NC
 H4   VDD   POWER
 H5   VSS   GND
 H6   VSS   GND
 H7   VSS   GND
 H8   VDD   POWER
 H9   NC   NC
 H10   NC   NC
 H11   ZZ   INBUF
 J1   DQB5   Progbuf1
 J2   NC   NC
 J3   VDDQ   POWER
 J4   VDD   POWER
 J5   VSS   GND
 J6   VSS   GND
 J7   VSS   GND
 J8   VDD   POWER
 J9   VDDQ   POWER
 J10   DQA4   Progbuf1
 J11   NC   NC
 K1   DQB6   Progbuf1
 K2   NC   NC
 K3   VDDQ   POWER
 K4   VDD   POWER
 K5   VSS   GND
 K6   VSS   GND
 K7   VSS   GND
 K8   VDD   POWER
 K9   VDDQ   POWER
 K10   DQA3   Progbuf1
 K11   NC   NC
 L1   DQB7   Progbuf1
 L2   NC   NC
 L3   VDDQ   POWER
 L4   VDD   POWER
 L5   VSS   GND
 L6   VSS   GND
 L7   VSS   GND
 L8   VDD   POWER
 L9   VDDQ   POWER
 L10   DQA2   Progbuf1
 L11   NC   NC
 M1   DQB8   Progbuf1
 M2   NC   NC
 M3   VDDQ   POWER
 M4   VDD   POWER
 M5   VSS   GND
 M6   VSS   GND
 M7   VSS   GND
 M8   VDD   POWER
 M9   VDDQ   POWER
 M10   DQA1   Progbuf1
 M11   NC   NC
 N1   DQPB   Progbuf1
 N2   NC   NC
 N3   VDDQ   POWER
 N4   VSS   GND
 N5   NC   NC
 N6   A18   INBUF
 N7   NC   NC
 N8   VSS   GND
 N9   VDDQ   POWER
 N10   NC   NC
 N11   NC   NC
 P1   NC   NC
 P2   NC   NC
 P3   A6   INBUF
 P4   A5   INBUF
 P5   TDI   INBUF
 P6   A1   INBUF
 P7   TDO   Progbuf2
 P8   A4   INBUF
 P9   A3   INBUF
 P10   A2   INBUF
 P11   A17   INBUF
 R1   LBO#   INBUF
 R2   A19   INBUF
 R3   A12   INBUF
 R4   A11   INBUF
 R5   TMS   INBUF
 R6   A0   INBUF
 R7   TCK   INBUF
 R8   A10   INBUF
 R9   A9   INBUF
 R10   A8   INBUF
 R11   A7   INBUF
[Component]   GS8321E32E
[Manufacturer]   GSI Technology
[Package]
|  variable   typ   min   max
R_pkg   0.2   0.1   0.5
L_pkg   3nH   1nH   5nH
C_pkg   1.5pF   1pF   3pF
[Pin]   signal_name model_name  R_pin   L_pin   C_pin
 A1   NC   NC
 A2   A14   INBUF
 A3   E1#   INBUF
 A4   BC#   INBUF
 A5   BB#   INBUF
 A6   E3#   INBUF
 A7   BW#   INBUF
 A8   ADSC#   INBUF
 A9   ADV#   INBUF
 A10   A13   INBUF
 A11   NC   NC
 B1   NC   NC
 B2   A16   INBUF
 B3   E2   INBUF
 B4   BD#   INBUF
 B5   BA#   INBUF
 B6   CK   INBUF
 B7   GW#   INBUF
 B8   G#   INBUF
 B9   ADSP   INBUF
 B10   A15   INBUF
 B11   NC   NC
 C1   NC   NC
 C2   NC   NC
 C3   VDDQ   POWER
 C4   VSS   GND
 C5   VSS   GND
 C6   VSS   GND
 C7   VSS   GND
 C8   VSS   GND
 C9   VDDQ   POWER
 C10   NC   NC
 C11   NC   NC
 D1   DQC8   Progbuf1
 D2   DQC4   Progbuf1
 D3   VDDQ   POWER
 D4   VDD   POWER
 D5   VSS   GND
 D6   VSS   GND
 D7   VSS   GND
 D8   VDD   POWER
 D9   VDDQ   POWER
 D10   DQB4   Progbuf1
 D11   DQB8   Progbuf1
 E1   DQC7   Progbuf1
 E2   DQC3   Progbuf1
 E3   VDDQ   POWER
 E4   VDD   POWER
 E5   VSS   GND
 E6   VSS   GND
 E7   VSS   GND
 E8   VDD   POWER
 E9   VDDQ   POWER
 E10   DQB3   Progbuf1
 E11   DQB7   Progbuf1
 F1   DQC6   Progbuf1
 F2   DQC2   Progbuf1
 F3   VDDQ   POWER
 F4   VDD   POWER
 F5   VSS   GND
 F6   VSS   GND
 F7   VSS   GND
 F8   VDD   POWER
 F9   VDDQ   POWER
 F10   DQB2   Progbuf1
 F11   DQB6   Progbuf1
 G1   DQC5   Progbuf1
 G2   DQC1   Progbuf1
 G3   VDDQ   POWER
 G4   VDD   POWER
 G5   VSS   GND
 G6   VSS   GND
 G7   VSS   GND
 G8   VDD   POWER
 G9   VDDQ   POWER
 G10   DQB1   Progbuf1
 G11   DQB5   Progbuf1
 H1   FT#   INBUF
 H2   MCL   INBUF
 H3   NC   NC
 H4   VDD   POWER
 H5   VSS   GND
 H6   VSS   GND
 H7   VSS   GND
 H8   VDD   POWER
 H9   NC   NC
 H10   NC   NC
 H11   ZZ   INBUF
 J1   DQD5   Progbuf1
 J2   DQD1   Progbuf1
 J3   VDDQ   POWER
 J4   VDD   POWER
 J5   VSS   GND
 J6   VSS   GND
 J7   VSS   GND
 J8   VDD   POWER
 J9   VDDQ   POWER
 J10   DQA1   Progbuf1
 J11   DQA5   Progbuf1
 K1   DQD6   Progbuf1
 K2   DQD2   Progbuf1
 K3   VDDQ   POWER
 K4   VDD   POWER
 K5   VSS   GND
 K6   VSS   GND
 K7   VSS   GND
 K8   VDD   POWER
 K9   VDDQ   POWER
 K10   DQA2   Progbuf1
 K11   DQA6   Progbuf1
 L1   DQD7   Progbuf1
 L2   DQD3   Progbuf1
 L3   VDDQ   POWER
 L4   VDD   POWER
 L5   VSS   GND
 L6   VSS   GND
 L7   VSS   GND
 L8   VDD   POWER
 L9   VDDQ   POWER
 L10   DQA3   Progbuf1
 L11   DQA7   Progbuf1
 M1   DQD8   Progbuf1
 M2   DQD4   Progbuf1
 M3   VDDQ   POWER
 M4   VDD   POWER
 M5   VSS   GND
 M6   VSS   GND
 M7   VSS   GND
 M8   VDD   POWER
 M9   VDDQ   POWER
 M10   DQA4   Progbuf1
 M11   DQA8   Progbuf1
 N1   NC   NC
 N2   NC   NC
 N3   VDDQ   POWER
 N4   VSS   GND
 N5   NC   NC
 N6   A18   INBUF
 N7   NC   NC
 N8   VSS   GND
 N9   VDDQ   POWER
 N10   NC   NC
 N11   NC   NC
 P1   NC   NC
 P2   NC   NC
 P3   A6   INBUF
 P4   A5   INBUF
 P5   TDI   INBUF
 P6   A1   INBUF
 P7   TDO   Progbuf2
 P8   A4   INBUF
 P9   A3   INBUF
 P10   A2   INBUF
 P11   A17   INBUF
 R1   LBO#   INBUF
 R2   A19   INBUF
 R3   A12   INBUF
 R4   A11   INBUF
 R5   TMS   INBUF
 R6   A0   INBUF
 R7   TCK   INBUF
 R8   A10   INBUF
 R9   A9   INBUF
 R10   A8   INBUF
 R11   A7   INBUF
[Component]   GS8321E36E
[Manufacturer]   GSI Technology
[Package]
|  variable   typ   min   max
R_pkg   0.2   0.1   0.5
L_pkg   3nH   1nH   5nH
C_pkg   1.5pF   1pF   3pF
[Pin]   signal_name model_name  R_pin   L_pin   C_pin
 A1   NC   NC
 A2   A14   INBUF
 A3   E1#   INBUF
 A4   BC#   INBUF
 A5   BB#   INBUF
 A6   E3#   INBUF
 A7   BW#   INBUF
 A8   ADSC#   INBUF
 A9   ADV#   INBUF
 A10   A13   INBUF
 A11   NC   NC
 B1   NC   NC
 B2   A16   INBUF
 B3   E2   INBUF
 B4   BD#   INBUF
 B5   BA#   INBUF
 B6   CK   INBUF
 B7   GW#   INBUF
 B8   G#   INBUF
 B9   ADSP   INBUF
 B10   A15   INBUF
 B11   NC   NC
 C1   DQPC   Progbuf1
 C2   NC   NC
 C3   VDDQ   POWER
 C4   VSS   GND
 C5   VSS   GND
 C6   VSS   GND
 C7   VSS   GND
 C8   VSS   GND
 C9   VDDQ   POWER
 C10   NC   NC
 C11   DQPB   Progbuf1
 D1   DQC8   Progbuf1
 D2   DQC4   Progbuf1
 D3   VDDQ   POWER
 D4   VDD   POWER
 D5   VSS   GND
 D6   VSS   GND
 D7   VSS   GND
 D8   VDD   POWER
 D9   VDDQ   POWER
 D10   DQB4   Progbuf1
 D11   DQB8   Progbuf1
 E1   DQC7   Progbuf1
 E2   DQC3   Progbuf1
 E3   VDDQ   POWER
 E4   VDD   POWER
 E5   VSS   GND
 E6   VSS   GND
 E7   VSS   GND
 E8   VDD   POWER
 E9   VDDQ   POWER
 E10   DQB3   Progbuf1
 E11   DQB7   Progbuf1
 F1   DQC6   Progbuf1
 F2   DQC2   Progbuf1
 F3   VDDQ   POWER
 F4   VDD   POWER
 F5   VSS   GND
 F6   VSS   GND
 F7   VSS   GND
 F8   VDD   POWER
 F9   VDDQ   POWER
 F10   DQB2   Progbuf1
 F11   DQB6   Progbuf1
 G1   DQC5   Progbuf1
 G2   DQC1   Progbuf1
 G3   VDDQ   POWER
 G4   VDD   POWER
 G5   VSS   GND
 G6   VSS   GND
 G7   VSS   GND
 G8   VDD   POWER
 G9   VDDQ   POWER
 G10   DQB1   Progbuf1
 G11   DQB5   Progbuf1
 H1   FT#   INBUF
 H2   MCL   INBUF
 H3   NC   NC
 H4   VDD   POWER
 H5   VSS   GND
 H6   VSS   GND
 H7   VSS   GND
 H8   VDD   POWER
 H9   NC   NC
 H10   NC   NC
 H11   ZZ   INBUF
 J1   DQD5   Progbuf1
 J2   DQD1   Progbuf1
 J3   VDDQ   POWER
 J4   VDD   POWER
 J5   VSS   GND
 J6   VSS   GND
 J7   VSS   GND
 J8   VDD   POWER
 J9   VDDQ   POWER
 J10   DQA1   Progbuf1
 J11   DQA5   Progbuf1
 K1   DQD6   Progbuf1
 K2   DQD2   Progbuf1
 K3   VDDQ   POWER
 K4   VDD   POWER
 K5   VSS   GND
 K6   VSS   GND
 K7   VSS   GND
 K8   VDD   POWER
 K9   VDDQ   POWER
 K10   DQA2   Progbuf1
 K11   DQA6   Progbuf1
 L1   DQD7   Progbuf1
 L2   DQD3   Progbuf1
 L3   VDDQ   POWER
 L4   VDD   POWER
 L5   VSS   GND
 L6   VSS   GND
 L7   VSS   GND
 L8   VDD   POWER
 L9   VDDQ   POWER
 L10   DQA3   Progbuf1
 L11   DQA7   Progbuf1
 M1   DQD8   Progbuf1
 M2   DQD4   Progbuf1
 M3   VDDQ   POWER
 M4   VDD   POWER
 M5   VSS   GND
 M6   VSS   GND
 M7   VSS   GND
 M8   VDD   POWER
 M9   VDDQ   POWER
 M10   DQA4   Progbuf1
 M11   DQA8   Progbuf1
 N1   DQPD   Progbuf1
 N2   NC   NC
 N3   VDDQ   POWER
 N4   VSS   GND
 N5   NC   NC
 N6   A18   INBUF
 N7   NC   NC
 N8   VSS   GND
 N9   VDDQ   POWER
 N10   NC   NC
 N11   DQPA   Progbuf1
 P1   NC   NC
 P2   NC   NC
 P3   A6   INBUF
 P4   A5   INBUF
 P5   TDI   INBUF
 P6   A1   INBUF
 P7   TDO   Progbuf2
 P8   A4   INBUF
 P9   A3   INBUF
 P10   A2   INBUF
 P11   A17   INBUF
 R1   LBO#   INBUF
 R2   A19   INBUF
 R3   A12   INBUF
 R4   A11   INBUF
 R5   TMS   INBUF
 R6   A0   INBUF
 R7   TCK   INBUF
 R8   A10   INBUF
 R9   A9   INBUF
 R10   A8   INBUF
 R11   A7   INBUF
[Component]   GS832218B
[Manufacturer]   GSI Technology
[Package]
|  variable   typ   min   max
R_pkg   0.2   0.1   0.5
L_pkg   3nH   1nH   5nH
C_pkg   1.5pF   1pF   3pF
[Pin]   signal_name model_name  R_pin   L_pin   C_pin
 A1   VDDQ   POWER
 A2   A6   INBUF
 A3   A7   INBUF
 A4   ADSP#   INBUF
 A5   A8   INBUF
 A6   A9   INBUF
 A7   VDDQ   POWER
 B1   NC   NC
 B2   A18   INBUF
 B3   A4   INBUF
 B4   ADSC#   INBUF
 B5   A15   INBUF
 B6   A17   INBUF
 B7   NC   NC
 C1   NC   NC
 C2   A5   INBUF
 C3   A3   INBUF
 C4   VDD   POWER
 C5   A14   INBUF
 C6   A16   INBUF
 C7   NC   NC
 D1   DQB1   Progbuf1
 D2   NC   NC
 D3   VSS   GND
 D4   ZQ   INBUF
 D5   VSS   GND
 D6   DQA9   Progbuf1
 D7   NC   NC
 E1   NC   NC
 E2   DQB2   Progbuf1
 E3   VSS   GND
 E4   E1#   INBUF
 E5   VSS   GND
 E6   NC   NC
 E7   DQA8   Progbuf1
 F1   VDDQ   POWER
 F2   NC   NC
 F3   VSS   GND
 F4   G#   INBUF
 F5   VSS   GND
 F6   DQA7   Progbuf1
 F7   VDDQ   POWER
 G1   NC   NC
 G2   DQB3   Progbuf1
 G3   BB#   INBUF
 G4   ADV#   INBUF
 G5   NC   NC
 G6   NC   NC
 G7   DQA6   Progbuf1
 H1   DQB4   Progbuf1
 H2   NC   NC
 H3   VSS   GND
 H4   GW#   INBUF
 H5   VSS   GND
 H6   DQA5   Progbuf1
 H7   NC   NC
 J1   VDDQ   POWER
 J2   VDD   POWER
 J3   NC   NC
 J4   VDD   POWER
 J5   NC   NC
 J6   VDD   POWER
 J7   VDDQ   POWER
 K1   NC   NC
 K2   DQB5   Progbuf1
 K3   VSS   GND
 K4   CK   INBUF
 K5   VSS   GND
 K6   NC   NC
 K7   DQA4   Progbuf1
 L1   DQB6   Progbuf1
 L2   NC   NC
 L3   NC   NC
 L4   SCD   INBUF
 L5   BA#   INBUF
 L6   DQA3   Progbuf1
 L7   NC   NC
 M1   VDDQ   POWER
 M2   DQB7   Progbuf1
 M3   VSS   GND
 M4   BW#   INBUF
 M5   VSS   GND
 M6   NC   NC
 M7   VDDQ   POWER
 N1   DQB8   Progbuf1
 N2   NC   NC
 N3   VSS   GND
 N4   A1   INBUF
 N5   VSS   GND
 N6   DQA2   Progbuf1
 N7   NC   NC
 P1   NC   NC
 P2   DQB9   Progbuf1
 P3   VSS   GND
 P4   A0   INBUF
 P5   VSS   GND
 P6   NC   NC
 P7   DQA1   Progbuf1
 R1   NC   NC
 R2   A2   INBUF
 R3   LBO#   INBUF
 R4   VDD   POWER
 R5   FT#   INBUF
 R6   A13   INBUF
 R7   NC   NC
 T1   NC   NC
 T2   A10   INBUF
 T3   A11   INBUF
 T4   A20   INBUF
 T5   A12   INBUF
 T6   A19   INBUF
 T7   ZZ   INBUF
 U1   VDDQ   POWER
 U2   TMS   INBUF
 U3   TDI   INBUF
 U4   TCK   INBUF
 U5   TDO   Progbuf2
 U6   NC   NC
 U7   VDDQ   POWER
[Component]   GS832236B
[Manufacturer]   GSI Technology
[Package]
|  variable   typ   min   max
R_pkg   0.2   0.1   0.5
L_pkg   3nH   1nH   5nH
C_pkg   1.5pF   1pF   3pF
[Pin]   signal_name model_name  R_pin   L_pin   C_pin
 A1   VDDQ   POWER
 A2   A6   INBUF
 A3   A7   INBUF
 A4   ADSP#   INBUF
 A5   A8   INBUF
 A6   A9   INBUF
 A7   VDDQ   POWER
 B1   NC   NC
 B2   A18   INBUF
 B3   A4   INBUF
 B4   ADSC#   INBUF
 B5   A15   INBUF
 B6   A17   INBUF
 B7   NC   NC
 C1   NC   NC
 C2   A5   INBUF
 C3   A3   INBUF
 C4   VDD   POWER
 C5   A14   INBUF
 C6   A16   INBUF
 C7   NC   NC
 D1   DQc4   Progbuf1
 D2   DQC9   Progbuf1
 D3   VSS   GND
 D4   ZQ   INBUF
 D5   VSS   GND
 D6   DQB9   Progbuf1
 D7   DQB4   Progbuf1
 E1   DQc3   Progbuf1
 E2   DQC8   Progbuf1
 E3   VSS   GND
 E4   E1#   INBUF
 E5   VSS   GND
 E6   DQB8   Progbuf1
 E7   DQB3   Progbuf1
 F1   VDDQ   POWER
 F2   DQC7   Progbuf1
 F3   VSS   GND
 F4   G#   INBUF
 F5   VSS   GND
 F6   DQB7   Progbuf1
 F7   VDDQ   POWER
 G1   DQc2   Progbuf1
 G2   DQC6   Progbuf1
 G3   BC#   INBUF
 G4   ADV#   INBUF
 G5   BB#   INBUF
 G6   DQB6   Progbuf1
 G7   DQB2   Progbuf1
 H1   DQc1   Progbuf1
 H2   DQC5   Progbuf1
 H3   VSS   GND
 H4   GW#   INBUF
 H5   VSS   GND
 H6   DQB5   Progbuf1
 H7   DQB1   Progbuf1
 J1   VDDQ   POWER
 J2   VDD   POWER
 J3   NC   NC
 J4   VDD   POWER
 J5   NC   NC
 J6   VDD   POWER
 J7   VDDQ   POWER
 K1   DQD1   Progbuf1
 K2   DQD5   Progbuf1
 K3   VSS   GND
 K4   CK   INBUF
 K5   VSS   GND
 K6   DQA5   Progbuf1
 K7   DQA1   Progbuf1
 L1   DQD2   Progbuf1
 L2   DQD6   Progbuf1
 L3   BD#   INBUF
 L4   SCD   INBUF
 L5   BA#   INBUF
 L6   DQA6   Progbuf1
 L7   DQA2   Progbuf1
 M1   VDDQ   POWER
 M2   DQD7   Progbuf1
 M3   VSS   GND
 M4   BW#   INBUF
 M5   VSS   GND
 M6   DQA7   Progbuf1
 M7   VDDQ   POWER
 N1   DQD3   Progbuf1
 N2   DQD8   Progbuf1
 N3   VSS   GND
 N4   A1   INBUF
 N5   VSS   GND
 N6   DQA8   Progbuf1
 N7   DQA3   Progbuf1
 P1   DQD4   Progbuf1
 P2   DQD9   Progbuf1
 P3   VSS   GND
 P4   A0   INBUF
 P5   VSS   GND
 P6   DQA9   Progbuf1
 P7   DQA4   Progbuf1
 R1   NC   NC
 R2   A2   INBUF
 R3   LBO#   INBUF
 R4   VDD   POWER
 R5   FT#   INBUF
 R6   A13   INBUF
 R7   NC   NC
 T1   NC   NC
 T2   NC   NC
 T3   A10   INBUF
 T4   A11   INBUF
 T5   A12   INBUF
 T6   A20   INBUF
 T7   ZZ   INBUF
 U1   VDDQ   POWER
 U2   TMS   INBUF
 U3   TDI   INBUF
 U4   TCK   INBUF
 U5   TDO   Progbuf2
 U6   NC   NC
 U7   VDDQ   POWER
[Component]   GS832218E
[Manufacturer]   GSI Technology
[Package]
|  variable   typ   min   max
R_pkg   0.2   0.1   0.5
L_pkg   3nH   1nH   5nH
C_pkg   1.5pF   1pF   3pF
[Pin]   signal_name model_name  R_pin   L_pin   C_pin
 A1   NC   NC
 A2   A14   INBUF
 A3   E1#   INBUF
 A4   BB#   INBUF
 A5   NC   NC
 A6   E3#   INBUF
 A7   BW#   INBUF
 A8   ADSC#   INBUF
 A9   ADV#   INBUF
 A10   A13   INBUF
 A11   A20   INBUF
 B1   NC   NC
 B2   A16   INBUF
 B3   E2   INBUF
 B4   NC   NC
 B5   BA#   INBUF
 B6   CK   INBUF
 B7   GW#   INBUF
 B8   G#   INBUF
 B9   ADSP   INBUF
 B10   A15   INBUF
 B11   NC   NC
 C1   NC   NC
 C2   NC   NC
 C3   VDDQ   POWER
 C4   VSS   GND
 C5   VSS   GND
 C6   VSS   GND
 C7   VSS   GND
 C8   VSS   GND
 C9   VDDQ   POWER
 C10   NC   NC
 C11   DQPA   Progbuf1
 D1   NC   NC
 D2   DQB1   Progbuf1
 D3   VDDQ   POWER
 D4   VDD   POWER
 D5   VSS   GND
 D6   VSS   GND
 D7   VSS   GND
 D8   VDD   POWER
 D9   VDDQ   POWER
 D10   NC   NC
 D11   DQA8   Progbuf1
 E1   NC   NC
 E2   DQB2   Progbuf1
 E3   VDDQ   POWER
 E4   VDD   POWER
 E5   VSS   GND
 E6   VSS   GND
 E7   VSS   GND
 E8   VDD   POWER
 E9   VDDQ   POWER
 E10   NC   NC
 E11   DQA7   Progbuf1
 F1   NC   NC
 F2   DQB3   Progbuf1
 F3   VDDQ   POWER
 F4   VDD   POWER
 F5   VSS   GND
 F6   VSS   GND
 F7   VSS   GND
 F8   VDD   POWER
 F9   VDDQ   POWER
 F10   NC   NC
 F11   DQA6   Progbuf1
 G1   NC   NC
 G2   DQB4   Progbuf1
 G3   VDDQ   POWER
 G4   VDD   POWER
 G5   VSS   GND
 G6   VSS   GND
 G7   VSS   GND
 G8   VDD   POWER
 G9   VDDQ   POWER
 G10   NC   NC
 G11   DQA5   Progbuf1
 H1   FT#   INBUF
 H2   MCL   INBUF
 H3   NC   NC
 H4   VDD   POWER
 H5   VSS   GND
 H6   VSS   GND
 H7   VSS   GND
 H8   VDD   POWER
 H9   NC   NC
 H10   ZQ   INBUF
 H11   ZZ   INBUF
 J1   DQB5   Progbuf1
 J2   NC   NC
 J3   VDDQ   POWER
 J4   VDD   POWER
 J5   VSS   GND
 J6   VSS   GND
 J7   VSS   GND
 J8   VDD   POWER
 J9   VDDQ   POWER
 J10   DQA4   Progbuf1
 J11   NC   NC
 K1   DQB6   Progbuf1
 K2   NC   NC
 K3   VDDQ   POWER
 K4   VDD   POWER
 K5   VSS   GND
 K6   VSS   GND
 K7   VSS   GND
 K8   VDD   POWER
 K9   VDDQ   POWER
 K10   DQA3   Progbuf1
 K11   NC   NC
 L1   DQB7   Progbuf1
 L2   NC   NC
 L3   VDDQ   POWER
 L4   VDD   POWER
 L5   VSS   GND
 L6   VSS   GND
 L7   VSS   GND
 L8   VDD   POWER
 L9   VDDQ   POWER
 L10   DQA2   Progbuf1
 L11   NC   NC
 M1   DQB8   Progbuf1
 M2   NC   NC
 M3   VDDQ   POWER
 M4   VDD   POWER
 M5   VSS   GND
 M6   VSS   GND
 M7   VSS   GND
 M8   VDD   POWER
 M9   VDDQ   POWER
 M10   DQA1   Progbuf1
 M11   NC   NC
 N1   DQPB   Progbuf1
 N2   SCD   INBUF
 N3   VDDQ   POWER
 N4   VSS   GND
 N5   NC   NC
 N6   A18   INBUF
 N7   NC   NC
 N8   VSS   GND
 N9   VDDQ   POWER
 N10   NC   NC
 N11   NC   NC
 P1   NC   NC
 P2   NC   NC
 P3   A6   INBUF
 P4   A5   INBUF
 P5   TDI   INBUF
 P6   A1   INBUF
 P7   TDO   Progbuf2
 P8   A4   INBUF
 P9   A3   INBUF
 P10   A2   INBUF
 P11   A17   INBUF
 R1   LBO#   INBUF
 R2   A19   INBUF
 R3   A12   INBUF
 R4   A11   INBUF
 R5   TMS   INBUF
 R6   A0   INBUF
 R7   TCK   INBUF
 R8   A10   INBUF
 R9   A9   INBUF
 R10   A8   INBUF
 R11   A7   INBUF
[Component]   GS832236E
[Manufacturer]   GSI Technology
[Package]
|  variable   typ   min   max
R_pkg   0.2   0.1   0.5
L_pkg   3nH   1nH   5nH
C_pkg   1.5pF   1pF   3pF
[Pin]   signal_name model_name  R_pin   L_pin   C_pin
 A1   NC   NC
 A2   A14   INBUF
 A3   E1#   INBUF
 A4   BC#   INBUF
 A5   BB#   INBUF
 A6   E3#   INBUF
 A7   BW#   INBUF
 A8   ADSC#   INBUF
 A9   ADV#   INBUF
 A10   A13   INBUF
 A11   NC   NC
 B1   NC   NC
 B2   A16   INBUF
 B3   E2   INBUF
 B4   BD#   INBUF
 B5   BA#   INBUF
 B6   CK   INBUF
 B7   GW#   INBUF
 B8   G#   INBUF
 B9   ADSP   INBUF
 B10   A15   INBUF
 B11   NC   NC
 C1   DQPC   Progbuf1
 C2   NC   NC
 C3   VDDQ   POWER
 C4   VSS   GND
 C5   VSS   GND
 C6   VSS   GND
 C7   VSS   GND
 C8   VSS   GND
 C9   VDDQ   POWER
 C10   NC   NC
 C11   DQPB   Progbuf1
 D1   DQC8   Progbuf1
 D2   DQC4   Progbuf1
 D3   VDDQ   POWER
 D4   VDD   POWER
 D5   VSS   GND
 D6   VSS   GND
 D7   VSS   GND
 D8   VDD   POWER
 D9   VDDQ   POWER
 D10   DQB4   Progbuf1
 D11   DQB8   Progbuf1
 E1   DQC7   Progbuf1
 E2   DQC3   Progbuf1
 E3   VDDQ   POWER
 E4   VDD   POWER
 E5   VSS   GND
 E6   VSS   GND
 E7   VSS   GND
 E8   VDD   POWER
 E9   VDDQ   POWER
 E10   DQB3   Progbuf1
 E11   DQB7   Progbuf1
 F1   DQC6   Progbuf1
 F2   DQC2   Progbuf1
 F3   VDDQ   POWER
 F4   VDD   POWER
 F5   VSS   GND
 F6   VSS   GND
 F7   VSS   GND
 F8   VDD   POWER
 F9   VDDQ   POWER
 F10   DQB2   Progbuf1
 F11   DQB6   Progbuf1
 G1   DQC5   Progbuf1
 G2   DQC1   Progbuf1
 G3   VDDQ   POWER
 G4   VDD   POWER
 G5   VSS   GND
 G6   VSS   GND
 G7   VSS   GND
 G8   VDD   POWER
 G9   VDDQ   POWER
 G10   DQB1   Progbuf1
 G11   DQB5   Progbuf1
 H1   FT#   INBUF
 H2   MCL   INBUF
 H3   NC   NC
 H4   VDD   POWER
 H5   VSS   GND
 H6   VSS   GND
 H7   VSS   GND
 H8   VDD   POWER
 H9   NC   NC
 H10   ZQ   INBUF
 H11   ZZ   INBUF
 J1   DQD5   Progbuf1
 J2   DQD1   Progbuf1
 J3   VDDQ   POWER
 J4   VDD   POWER
 J5   VSS   GND
 J6   VSS   GND
 J7   VSS   GND
 J8   VDD   POWER
 J9   VDDQ   POWER
 J10   DQA1   Progbuf1
 J11   DQA5   Progbuf1
 K1   DQD6   Progbuf1
 K2   DQD2   Progbuf1
 K3   VDDQ   POWER
 K4   VDD   POWER
 K5   VSS   GND
 K6   VSS   GND
 K7   VSS   GND
 K8   VDD   POWER
 K9   VDDQ   POWER
 K10   DQA2   Progbuf1
 K11   DQA6   Progbuf1
 L1   DQD7   Progbuf1
 L2   DQD3   Progbuf1
 L3   VDDQ   POWER
 L4   VDD   POWER
 L5   VSS   GND
 L6   VSS   GND
 L7   VSS   GND
 L8   VDD   POWER
 L9   VDDQ   POWER
 L10   DQA3   Progbuf1
 L11   DQA7   Progbuf1
 M1   DQD8   Progbuf1
 M2   DQD4   Progbuf1
 M3   VDDQ   POWER
 M4   VDD   POWER
 M5   VSS   GND
 M6   VSS   GND
 M7   VSS   GND
 M8   VDD   POWER
 M9   VDDQ   POWER
 M10   DQA4   Progbuf1
 M11   DQA8   Progbuf1
 N1   DQPD   Progbuf1
 N2   SCD   INBUF
 N3   VDDQ   POWER
 N4   VSS   GND
 N5   NC   NC
 N6   A18   INBUF
 N7   NC   NC
 N8   VSS   GND
 N9   VDDQ   POWER
 N10   NC   NC
 N11   DQPA   Progbuf1
 P1   NC   NC
 P2   NC   NC
 P3   A6   INBUF
 P4   A5   INBUF
 P5   TDI   INBUF
 P6   A1   INBUF
 P7   TDO   Progbuf2
 P8   A4   INBUF
 P9   A3   INBUF
 P10   A2   INBUF
 P11   A17   INBUF
 R1   LBO#   INBUF
 R2   A19   INBUF
 R3   A12   INBUF
 R4   A11   INBUF
 R5   TMS   INBUF
 R6   A0   INBUF
 R7   TCK   INBUF
 R8   A10   INBUF
 R9   A9   INBUF
 R10   A8   INBUF
 R11   A7   INBUF
[Component]   GS8320Z18T
[Manufacturer]   GSI Technology
[Package]
|  variable   typ   min   max
R_pkg   0.2   0.1   0.5
L_pkg   3nH   1nH   5nH
C_pkg   1.5pF   1pF   3pF
[Pin]   signal_name model_name  R_pin   L_pin   C_pin
 1   NC   NC
 2   NC   NC
 3   NC   NC
 4   VDDQ   POWER
 5   VSS   GND
 6   NC   NC
 7   NC   NC
 8   DQB1   Progbuf1
 9   DQB2   Progbuf1
 10   VSS   GND
 11   VDDQ   POWER
 12   DQB3   Progbuf1
 13   DQB4   Progbuf1
 14   FT#   INBUF
 15   VDD   POWER
 16   NC   NC
 17   VSS   GND
 18   DQB5   Progbuf1
 19   DQB6   Progbuf1
 20   VDDQ   POWER
 21   VSS   GND
 22   DQB7   Progbuf1
 23   DQB8   Progbuf1
 24   DQB9   Progbuf1
 25   NC   NC
 26   VSS   GND
 27   VDDQ   POWER
 28   NC   NC
 29   NC   NC
 30   NC   NC
 31   LBO#   INBUF
 32   A5   INBUF
 33   A4   INBUF
 34   A3   INBUF
 35   A2   INBUF
 36   A1   INBUF
 37   A0   INBUF
 38   NC   NC
 39   NC   NC
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| Models and submodels in the file (18): VIO_2Ldriver (I/O), VIO_2Hdriver (I/O), VIO_3Ldriver (I/O), VIO_3Hdriver (I/O), VIO_4Ldriver (I/O), VIO_4Hdriver (I/O), VIO_5Ldriver (I/O), VIO_5Hdriver (I/O), VIO_6Ldriver (I/O), VIO_6Hdriver (I/O), TDO_2driver (3-state), TDO_3driver (3-state), TDO_4driver (3-state), TDO_5driver (3-state), TDO_6driver (3-state), INBUF3_3 (Input), INBUF2_5 (Input), INBUF1_8 (Input)
